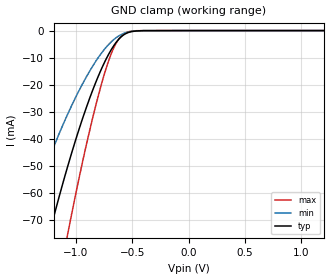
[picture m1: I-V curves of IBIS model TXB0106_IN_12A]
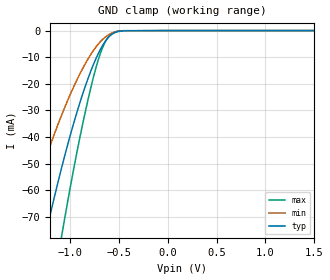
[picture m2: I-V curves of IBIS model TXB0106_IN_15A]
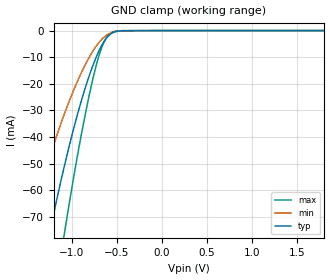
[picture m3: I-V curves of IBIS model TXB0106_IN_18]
| TEXAS INSTRUMENTS INCORPORATED
| Standard Linear and Logic Group
| IBIS Model of TXB0106
| 6-Bit Bidirectional Voltage-Level Translator with Auto Direction
| Sensing and +/-15-kV ESD Protect
| This file contains package information for the following:
|  TSSOP 16-pin (PW) package as [Component] TXB0106PWR
|  QFN 16-pin (RGY) package as [Component] TXB0106RGYR
| This device can be powered at the following Vccs:
|  1.2 volt Vcca
|  1.5 volt Vcca
|  1.8 volt Vcca
|  2.5 volt Vcca
|  3.3 volt Vcca
|  1.8 volt Vccb
|  2.5 volt Vccb
|  3.3 volt Vccb
|  5.0 volt Vccb
|  Vccb >= Vcca
| This file provides unique models under the [Model Selector] for each Vcc.
| For operation at a specific Vcc, select the appropriate model after each
| [Model Selector] keyword.
[IBIS Ver]   3.2
[Comment char]  |_char
[File Name]   txb0106.ibs
[File Rev]   1.0
[Date]   April 5, 2013
[Source]   Data created from TI-SPICE simulations at TI-SLL.
[Notes]   The following is an IBIS list for the TXB0106.
   Please contact sllibis@ti.com with questions and
   comments concerning SLL IBIS models.
   - As there is no power clamp diode we removed the Power Clamp
   table data from the IN and I/O Models.
   - IBIS 3.2 SYNTAX CANNOT DESCRIBE THE CHARACTERISTICS OF
   ANY OUTPUT STRUCTURES THAT DYNAMICALLY CHANGES THE
   IMPEDANCES DURING THE TRANSITION. THIS DEVICE USE SIMILAR
   OUTPUT STRUCTURE AND THEREFORE THE SIMULATION RESULTS
   MAY NOT BE ACCURATE. TI RECOMMENDS THE USE OF SPICE
   SIMULATION WHEN SIMULATION ACCURACY IS IMPORTANT.
[Disclaimer] Property of Texas Instruments Incorporated.  Unauthorized
   reproduction and/or distribution is strictly prohibited.
   This product is protected under copyright law.
   Created  2013, (C) Copyright  2013, Texas Instruments
   Incorporated, All Rights Reserved
   UNLESS THERE IS A SIGNED, WRITTEN AGREEMENT TO THE
   CONTRARY, TEXAS INSTRUMENTS (TI) IS PROVIDING THE IBIS
   MODELS  AND WITHOUT ANY WARRANTY, EXPRESSED OR
   IMPLIED.  TI assumes no liability for:
   1) the accuracy of the IBIS models provided to your
   company;
   2) the proper functioning of these IBIS Models in your
   design or for any resulting applications; or
   3) infringement of patents, copyrights or intellectual
   property rights resulting from your use of these IBIS
   models.
   TI provides IBIS Models as a service to our customers.
   You and your company shall not distribute, sell or give
   these models to anyone else without prior written
   permission from TI.
   TI reserves the right to make changes to our products or
   to discontinue any semiconductor product or service
   without notice, and advises our customers to obtain the
   latest version of relevant information to verify, before
   placing orders, that the information being relied on is
   current.
   Please be aware that your receipt and use of the IBIS
   information provided shall serve as acceptance of these
   terms and conditions.  If you do not accept these terms,
   you should return or destroy the IBIS models and any
   other accompanying information immediately.
| Component TXB0106PWR 16-PIN TSSOP
[Component]   TXB0106PWR
[Manufacturer]   Texas Instruments, Inc.
[Package]
|   typ   min   max
R_pkg   0.22228   0.18337   0.26730
L_pkg   2.73510nH   2.34613nH   3.22072nH
C_pkg   0.42640pF   0.37822pF   0.51154pF
[Pin]   signal_name   model_name   R_pin   L_pin   C_pin
1   A1   TXB0106_IO_A   0.18337   2.98261nH   0.48201pF
2   VCCA   POWER   0.23036   2.91673nH   0.50176pF
3   A2   TXB0106_IO_A   0.22064   2.48044nH   0.37822pF
4   A3   TXB0106_IO_A   0.20469   2.34613nH   0.38084pF
5   A4   TXB0106_IO_A   0.21147   2.40261nH   0.38357pF
6   A5   TXB0106_IO_A   0.23867   2.63153nH   0.38509pF
7   A6   TXB0106_IO_A   0.26035   3.16332nH   0.50924pF
8   OE   TXB0106_IN   0.19042   3.04383nH   0.48315pF
9   GND   GND   0.19468   3.07823nH   0.48454pF
10   B6   TXB0106_IO_B   0.26730   3.22072nH   0.51154pF
11   B5   TXB0106_IO_B   0.24899   2.71663nH   0.38855pF
12   B4   TXB0106_IO_B   0.22374   2.50311nH   0.38779pF
13   B3   TXB0106_IO_B   0.21693   2.44623nH   0.38525pF
14   B2   TXB0106_IO_B   0.23139   2.56874nH   0.38214pF
15   VCCB   POWER   0.23733   2.97413nH   0.50515pF
16   B1   TXB0106_IO_B   0.19179   3.05051nH   0.48581pF
| Component TXB0106RGYR 16-PIN QFN
[Component]   TXB0106RGYR
[Manufacturer]   Texas Instruments, Inc.
[Package]
|   typ   min   max
R_pkg   0.07857   0.07015   0.09566
L_pkg   1.13887nH   1.00107nH   1.42705nH
C_pkg   0.22279pF   0.19820pF   0.24196pF
[Pin]   signal_name   model_name   R_pin   L_pin   C_pin
1   A1   TXB0106_IO_A   0.07149   1.02086nH   0.19820pF
2   VCCA   POWER   0.08214   1.20235nH   0.22263pF
3   A2   TXB0106_IO_A   0.07361   1.05833nH   0.22523pF
4   A3   TXB0106_IO_A   0.07015   1.00107nH   0.21152pF
5   A4   TXB0106_IO_A   0.07276   1.04443nH   0.21469pF
6   A5   TXB0106_IO_A   0.08066   1.17669nH   0.23399pF
7   A6   TXB0106_IO_A   0.09217   1.37286nH   0.24196pF
8   OE   TXB0106_IN   0.07530   1.08459nH   0.22029pF
9   GND   GND   0.07756   1.11893nH   0.21254pF
10   B6   TXB0106_IO_B   0.09566   1.42705nH   0.23533pF
11   B5   TXB0106_IO_B   0.08457   1.23603nH   0.23747pF
12   B4   TXB0106_IO_B   0.07740   1.11425nH   0.21915pF
13   B3   TXB0106_IO_B   0.07483   1.07083nH   0.21619pF
14   B2   TXB0106_IO_B   0.07782   1.12099nH   0.22962pF
15   VCCB   POWER   0.08581   1.25729nH   0.23649pF
16   B1   TXB0106_IO_B   0.07503   1.07734nH   0.21264pF
| Model TXB0106_IN
[Model Selector]   TXB0106_IN
TXB0106_IN_12A   1.2 volt Vcc
TXB0106_IN_15A   1.5 volt Vcc
TXB0106_IN_18   1.8 volt Vcc
TXB0106_IN_25   2.5 volt Vcc
TXB0106_IN_33   3.3 volt Vcc
| Model TXB0106_IO_B
[Model Selector]   TXB0106_IO_B
TXB0106_IO_B_18   1.8 volt Vcc
TXB0106_IO_B_25   2.5 volt Vcc
TXB0106_IO_B_33   3.3 volt Vcc
TXB0106_IO_B_50   5 volt Vcc
TXB0106_IO_B_OS_18   1.8 volt Vcc
TXB0106_IO_B_OS_25   2.5 volt Vcc
TXB0106_IO_B_OS_33   3.3 volt Vcc
TXB0106_IO_B_OS_50   5 volt Vcc
| Model TXB0106_IO_A
[Model Selector]   TXB0106_IO_A
TXB0106_IO_A_12A   1.2 volt Vcc
TXB0106_IO_A_15A   1.5 volt Vcc
TXB0106_IO_A_18   1.8 volt Vcc
TXB0106_IO_A_25   2.5 volt Vcc
TXB0106_IO_A_33   3.3 volt Vcc
TXB0106_IO_A_OS_12A   1.2 volt Vcc
TXB0106_IO_A_OS_15A   1.5 volt Vcc
TXB0106_IO_A_OS_18   1.8 volt Vcc
TXB0106_IO_A_OS_25   2.5 volt Vcc
TXB0106_IO_A_OS_33   3.3 volt Vcc
| Models and submodels in the file (23): TXB0106_IN_12A (Input), TXB0106_IN_15A (Input), TXB0106_IN_18 (Input), TXB0106_IN_25 (Input), TXB0106_IN_33 (Input), TXB0106_IO_B_18 (I/O), TXB0106_IO_B_25 (I/O), TXB0106_IO_B_33 (I/O), TXB0106_IO_B_50 (I/O), TXB0106_IO_B_OS_18 (I/O), TXB0106_IO_B_OS_25 (I/O), TXB0106_IO_B_OS_33 (I/O), TXB0106_IO_B_OS_50 (I/O), TXB0106_IO_A_12A (I/O), TXB0106_IO_A_15A (I/O), TXB0106_IO_A_18 (I/O), TXB0106_IO_A_25 (I/O), TXB0106_IO_A_33 (I/O), TXB0106_IO_A_OS_12A (I/O), TXB0106_IO_A_OS_15A (I/O), TXB0106_IO_A_OS_18 (I/O), TXB0106_IO_A_OS_25 (I/O), TXB0106_IO_A_OS_33 (I/O)
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[Model]   TXB0106_IN_12A
Model_type  Input
Vinl=0.42
Vinh=0.78
| variable   typ   min   max
C_comp   3.10pF   2.74pF   3.31pF
[Temperature Range]   40   100   -40
| Ambient temperature   25   85   -40
[Voltage range]   1.2   1.2   1.2
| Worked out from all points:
|   GND clamp passes 1 mA (typ) near -0.55 V on its own axis
[GND Clamp]
| TXB0104_IN_12A
|   Voltage   I(typ)   I(min)   I(max)
-5.5V     -1.044A    -792.2mA   -1.306A
-1.49V    -118.9mA   -76.3mA    -173.2mA
-1.445V   -110.7mA   -70.75mA   -161.9mA
-1.23V    -73.88mA   -46.23mA   -109.9mA
-1.075V   -50.27mA   -30.94mA   -75.32mA
-1.04V    -45.35mA   -27.8mA    -67.96mA
-905mV    -28.01mA   -16.85mA   -41.57mA
-770mV    -13.77mA   -8.095mA   -19.13mA
-670mV    -5.912mA   -3.496mA   -6.845mA
-580mV    -1.682mA   -1.115mA   -1.36mA
-405mV    -29.17uA   -32.54uA   -7.015uA
1.2V      84.13pA    453.1pA    9.863pA
[Model]   TXB0106_IN_15A
Model_type  Input
Vinl=0.49
Vinh=1.04
| variable   typ   min   max
C_comp   3.06pF   2.68pF   3.28pF
[Temperature Range]   40   100   -40
| Ambient temperature   25   85   -40
[Voltage range]   1.5   1.4   1.6
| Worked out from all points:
|   GND clamp passes 1 mA (typ) near -0.55 V on its own axis
[GND Clamp]
| TXB0104_IN_15A
|   Voltage   I(typ)   I(min)   I(max)
-5.5V     -1.044A    -792.2mA   -1.306A
-1.485V   -118mA     -75.68mA   -171.9mA
-1.255V   -77.94mA   -48.9mA    -115.7mA
-1.215V   -71.47mA   -44.66mA   -106.4mA
-1.095V   -53.15mA   -32.79mA   -79.61mA
-1.06V    -48.14mA   -29.58mA   -72.15mA
-895mV    -26.84mA   -16.12mA   -39.76mA
-760mV    -12.86mA   -7.552mA   -17.68mA
-665mV    -5.597mA   -3.318mA   -6.389mA
-575mV    -1.539mA   -1.032mA   -1.212mA
-450mV    -95.72uA   -91.06uA   -34.08uA
1.5V      97.95pA    495pA      11.19pA
[Model]   TXB0106_IN_18
Model_type  Input
Vinl=0.5775
Vinh=1.2675
| variable   typ   min   max
C_comp   3.03pF   2.64pF   3.31pF
[Temperature Range]   40   100   -40
| Ambient temperature   25   85   -40
[Voltage range]   1.8   1.65   1.95
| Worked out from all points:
|   GND clamp passes 1 mA (typ) near -0.55 V on its own axis
[GND Clamp]
| TXB0104_IN_18
|   Voltage   I(typ)   I(min)   I(max)
-5.5V     -1.044A    -792.2mA   -1.306A
-1.5V     -120.7mA   -77.56mA   -175.7mA
-1.45V    -111.6mA   -71.36mA   -163.1mA
-1.24V    -75.49mA   -47.29mA   -112.2mA
-1.08V    -50.99mA   -31.4mA    -76.39mA
-1.06V    -48.14mA   -29.58mA   -72.15mA
-920mV    -29.8mA    -17.97mA   -44.33mA
-765mV    -13.32mA   -7.821mA   -18.4mA
-660mV    -5.291mA   -3.146mA   -5.95mA
-575mV    -1.539mA   -1.032mA   -1.212mA
-435mV    -65.01uA   -65.03uA   -20.45uA
1.8V      112.9pA    537.9pA    13.45pA
